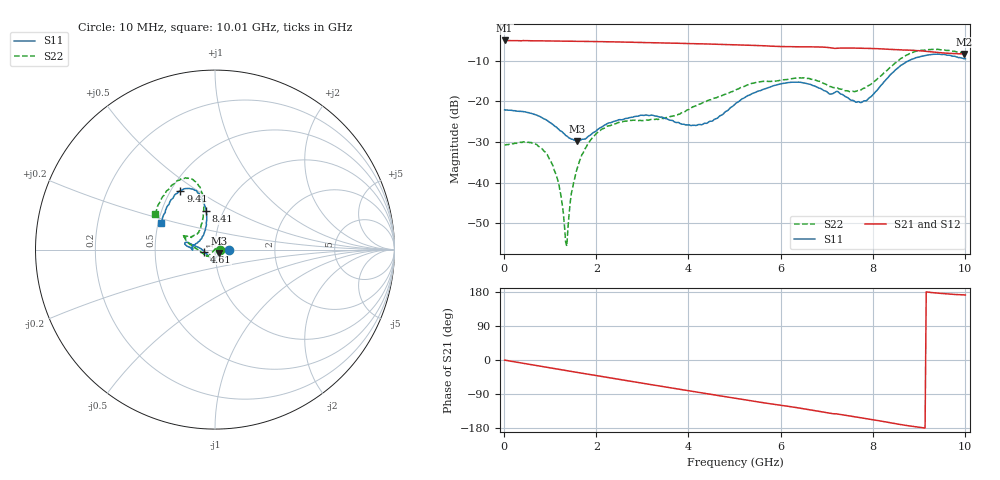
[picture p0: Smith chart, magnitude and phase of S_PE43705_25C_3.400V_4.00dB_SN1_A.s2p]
! Device ID: PE43705
! Serial: 1
! Insertion: A
! Impedance: 50 ohm
! Temp: 25C
! VDD: 3.400V
! Attenuation Step: 4.00dB
#  Hz  S  RI  R  50
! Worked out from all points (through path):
!   401 points, 10 MHz to 10.01 GHz, reference 50 ohm
!   highest |S21| = -5.00 dB at 10 MHz (marker M1); lowest = -8.3 dB at 9.985 GHz (marker M2)
!   group delay of S21, straight-line fit = 53.8 ps
!   lowest |S11| = -29.8 dB at 1.585 GHz (marker M3), VSWR 1.07, Z = 52.5 - j2.2 ohm
!   |S11| at or under -10 dB: start of sweep to 8.78 GHz
!   |S22| runs from -55.7 to -7.2 dB; largest |S21 - S12| = 0.005
!   S11 on the Smith chart (normalised r, x): 10 MHz: 1.17, -0.00; 4.61 GHz: 0.89, -0.02; 8.41 GHz: 0.83, +0.37; 9.41 GHz: 0.56, +0.43; 10.01 GHz: 0.52, +0.17
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1e7  0.0787 -0.00029  0.5625 -0.00263  0.5631 -0.00246  0.0293 7.14e-05
5.6e8  0.0703 0.0137  0.5454 -0.1137  0.5456 -0.1136  0.0253 0.018
9.1e8  0.0584 0.0101  0.5251 -0.1806  0.5252 -0.1801  0.0163 0.0162
1.16e9  0.0463 0.00155  0.5052 -0.2249  0.505 -0.2247  0.00657 0.00868
1.335e9  0.0373 -0.00738  0.4889 -0.2554  0.489 -0.2552  -0.00106 0.00151
1.385e9  0.035 -0.0099  0.484 -0.2641  0.4841 -0.264  -0.00273 -0.000548
1.485e9  0.0302 -0.0158  0.4734 -0.2808  0.4736 -0.2807  -0.00645 -0.00549
1.585e9  0.0245 -0.0209  0.4619 -0.2968  0.4622 -0.2967  -0.0109 -0.0102
1.685e9  0.0201 -0.0275  0.4507 -0.3125  0.4506 -0.3125  -0.0158 -0.0153
2.21e9  0.000471 -0.052  0.3808 -0.3862  0.381 -0.386  -0.0343 -0.0337
3.36e9  -0.0157 -0.0625  0.1936 -0.4883  0.1943 -0.4877  -0.0513 -0.0316
4.11e9  -0.0367 -0.0349  0.0611 -0.5105  0.0619 -0.5103  -0.0854 -0.0103
4.61e9  -0.0605 -0.0108  -0.0274 -0.5041  -0.0261 -0.5039  -0.1105 0.0094
5.01e9  -0.0913 0.0123  -0.0934 -0.4879  -0.0928 -0.4879  -0.1351 0.0267
5.985e9  -0.1582 0.0406  -0.2308 -0.4141  -0.2286 -0.4147  -0.1686 0.0659
6.685e9  -0.1566 0.0194  -0.3158 -0.3465  -0.3156 -0.3463  -0.1695 0.077
7.735e9  -0.076 0.0594  -0.4001 -0.2092  -0.3987 -0.2105  -0.085 0.1082
8.36e9  -0.0471 0.2009  -0.4234 -0.1128  -0.4222 -0.1147  -0.0634 0.2497
8.41e9  -0.0508 0.2143  -0.4233 -0.1048  -0.4225 -0.1059  -0.0649 0.2626
9.41e9  -0.1928 0.3289  -0.4001 0.0256  -0.3989 0.0251  -0.2124 0.3827
9.985e9  -0.2958 0.1552  -0.3803 0.0551  -0.3811 0.0546  -0.3284 0.2104
1.001e10  -0.3026 0.1456  -0.3816 0.0562  -0.3829 0.0554  -0.3363 0.199
